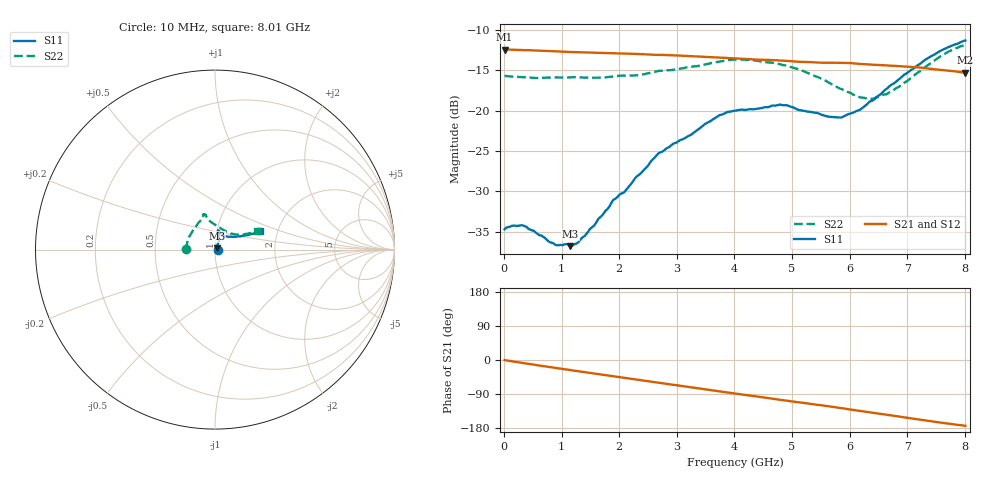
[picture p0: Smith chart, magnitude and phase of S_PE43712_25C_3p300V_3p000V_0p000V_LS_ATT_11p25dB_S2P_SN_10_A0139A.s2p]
! DEVICE ID: PE43712
! File Path: z:\PE43713\PE43713_CHAR_NOM_04292014\AMB\3p300\LS_ATT_11p25dB\PE43713_AMB_3p300V_3p000V_0p000V_LS_ATT_11p25dB_S2P_SN_10_A0139A.s2p
! Serial: 10
! Lot: A0139A
! Temp: 25C
! VDD: 3.300
! VSS: 0.000
! Control_Hi: 3.000
! Control_Lo: 0.000
! Attenuation Step: 11.25dB
! Port 1: RF1
! Port 2: RF2
! ThroughPath:1-2
! IDD: 0.0001471468
! ISS: -5.48e-008
#  Hz  S  RI  R  50
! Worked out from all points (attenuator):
!   801 points, 10 MHz to 8.01 GHz, reference 50 ohm
!   highest |S21| = -12.44 dB at 10 MHz (marker M1); lowest = -15.3 dB at 8.01 GHz (marker M2)
!   lowest |S11| = -36.8 dB at 1.15 GHz (marker M3), VSWR 1.03, Z = 51.2 + j0.851 ohm
!   |S11| at or under -10 dB: start of sweep to end of sweep
!   |S22| runs from -18.6 to -11.9 dB; largest |S21 - S12| = 0.00087
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1e7  0.0184 0.000276  0.2389 -0.00133  0.239 -0.00127  -0.1641 0.00111
3.3e8  0.0194 -4.26e-05  0.2345 -0.0333  0.2344 -0.0331  -0.1598 0.0194
9e8  0.0141 0.00423  0.2171 -0.0839  0.2172 -0.084  -0.1522 0.0502
1.15e9  0.0118 0.00831  0.2062 -0.1032  0.2063 -0.1034  -0.1474 0.0642
1.26e9  0.0116 0.00949  0.2012 -0.1113  0.2013 -0.1115  -0.1453 0.0694
1.35e9  0.0118 0.0111  0.1969 -0.118  0.1969 -0.118  -0.1423 0.0737
1.9e9  0.0134 0.0245  0.166 -0.154  0.166 -0.154  -0.1247 0.1049
2.1e9  0.0141 0.0283  0.1531 -0.1654  0.1531 -0.1653  -0.119 0.114
2.68e9  0.0224 0.0495  0.1114 -0.1911  0.1113 -0.1911  -0.0916 0.1503
3.72e9  0.0226 0.0898  0.0286 -0.211  0.0284 -0.211  -0.0652 0.1896
4.01e9  0.021 0.0978  0.00557 -0.2105  0.00553 -0.2104  -0.0641 0.1972
4.79e9  0.0185 0.1073  -0.0522 -0.1974  -0.0523 -0.1976  -0.0505 0.187
5.35e9  0.0292 0.0931  -0.0884 -0.1787  -0.0884 -0.1785  -0.0343 0.1634
5.64e9  0.0398 0.0824  -0.1053 -0.1676  -0.1053 -0.1677  -0.0141 0.1482
5.87e9  0.0502 0.0759  -0.1196 -0.157  -0.1195 -0.157  0.00531 0.1352
6.17e9  0.0703 0.0722  -0.1354 -0.1397  -0.1352 -0.1399  0.0357 0.1157
6.31e9  0.0839 0.0714  -0.1413 -0.1318  -0.141 -0.1319  0.0518 0.1067
6.42e9  0.0927 0.0712  -0.1457 -0.1254  -0.1455 -0.1254  0.0636 0.1001
6.68e9  0.1204 0.0722  -0.1557 -0.1088  -0.1554 -0.1089  0.0939 0.0885
7.36e9  0.1934 0.0848  -0.1716 -0.0609  -0.1715 -0.0609  0.1703 0.0872
7.72e9  0.2288 0.0948  -0.1725 -0.0364  -0.1724 -0.0365  0.2114 0.096
8.01e9  0.2501 0.1063  -0.1707 -0.0188  -0.1705 -0.019  0.2318 0.1009
